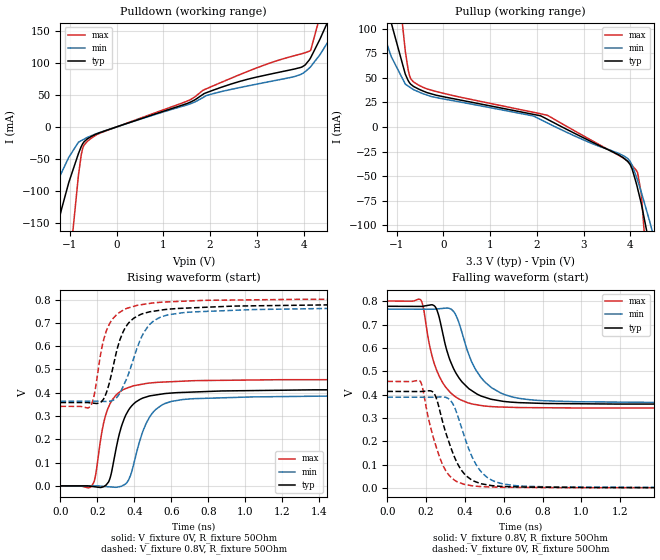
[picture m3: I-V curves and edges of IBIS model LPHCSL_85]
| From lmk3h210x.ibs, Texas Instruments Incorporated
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[Model]   LPHCSL_85
Model_type   Output
Polarity   Non-Inverting
Vmeas = 0.375
Vref = 0
Cref = 2pF
Rref = 100000
|   typ   min   max
C_comp   2.5pF   2pF   3pF
[Voltage Range]   3.3   3.135   3.465
[Temperature Range]   45   125   -40
[Pullup Reference]   3.3   3.135   3.465
[Pulldown Reference]   -0   -0   -0
[Power Clamp Reference]   3.3   3.135   3.465
[GND Clamp Reference]   0   0   0
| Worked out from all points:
|   slope of the pulldown table from 0 to 0.495 V, typ, clamps not added: 40.7 ohm
|   slope of the pullup table from 0 to 0.495 V, typ, clamps not added: 107 ohm
|   falling waveform, V_fixture 0.8V, R_fixture 50Ohm: 20-80 % time 123ps typ, 139ps min, 102ps max; typ from 0.779 V to 0.358 V
|   rising waveform, V_fixture 0V, R_fixture 50Ohm: 20-80 % time 90.9ps typ, 105ps min, 78.8ps max; typ from 0 V to 0.414 V
|   rising waveform, V_fixture 0.8V, R_fixture 50Ohm: 20-80 % time 99.8ps typ, 126ps min, 83.7ps max; typ from 0.358 V to 0.779 V
|   falling waveform, V_fixture 0V, R_fixture 50Ohm: 20-80 % time 106ps typ, 113ps min, 93.7ps max; typ from 0.414 V to 0 V
[Pulldown]
|   Voltage   I(typ)   I(min)   I(max)
-3.3V     -900mA     -529.4mA   -2.692A
-1.944V   -397.8mA   -215.8mA   -1.204A
-1.251V   -154.5mA   -84.31mA   -452.1mA
-1.023V   -86.95mA   -47.54mA   -227.5mA
-726mV    -26.52mA   -20.29mA   -33.92mA
-438.9mV  -11.27mA   -10.73mA   -12.68mA
3.977V    93.87mA    83.19mA    114.5mA
4.155V    108.2mA    94.14mA    119.8mA
4.353V    137mA      112.7mA    173mA
4.6V      177.5mA    141.8mA    276.7mA
4.927V    242.4mA    186.9mA    427.5mA
6.6V      632.4mA    489.5mA    1.311A
[Pullup]
|   Voltage   I(typ)   I(min)   I(max)
-3.3V     605.2mA    434.6mA    1.355A
-1.617V   212.4mA    144.7mA    463.6mA
-1.112V   105.1mA    71.14mA    210.1mA
-815.1mV  53.58mA    43.48mA    76.96mA
-726mV    44.97mA    40.66mA    52.4mA
-627mV    40.85mA    37.62mA    45.33mA
2.224V    7.749mA    4.058mA    11.86mA
3.937V    -34.84mA   -31.89mA   -34.65mA
4.155V    -62.59mA   -54.39mA   -46.61mA
4.372V    -111.3mA   -89.19mA   -155mA
4.491V    -145.8mA   -109.7mA   -248.9mA
6.6V      -933.8mA   -596.3mA   -2.548A
[Ramp]
R_load = 50
|   typ   min   max
dV/dt_r   0.248241/9.07181e-11   0.233324/1.04843e-10   0.27405/7.87855e-11
dV/dt_f   0.252877/1.21232e-10   0.242002/1.38069e-10   0.276271/1.01591e-10
[Falling Waveform]
V_fixture = 0.8V
V_fixture_min = 0.8V
V_fixture_max = 0.8V
R_fixture = 50Ohm
C_fixture = 0F
|   Time   V(typ)   V(min)   V(max)
0s        779.3mV    767mV      801.9mV
173.6ps   778.7mV    766.7mV    804.9mV
250.7ps   771.7mV    767.4mV    512.1mV
329.3ps   534.8mV    766.9mV    405.7mV
385.6ps   453.9mV    663.2mV    375.1mV
436.4ps   416.5mV    537.1mV    360.2mV
493.8ps   391.2mV    462.4mV    352mV
659.2ps   366.7mV    387.3mV    345.2mV
978.6ps   361mV      369.6mV    342.9mV
5ns       357.8mV    363.7mV    341.5mV
[Rising Waveform]
V_fixture = 0V
V_fixture_min = 0V
V_fixture_max = 0V
R_fixture = 50Ohm
C_fixture = 0F
|   Time   V(typ)   V(min)   V(max)
0s        161.5uV    251.5uV    87.97uV
173.6ps   -2.622mV   115.8uV    5.086mV
246.1ps   2.961mV    -2.859mV   306.9mV
271ps     40.38mV    -4.434mV   356.5mV
299.8ps   155.2mV    -5.936mV   389.1mV
368.1ps   325mV      24.64mV    422.2mV
465.5ps   382.2mV    271.2mV    440mV
549.7ps   394.6mV    347.8mV    445.6mV
720.7ps   403.1mV    374.4mV    451.7mV
5ns       413.9mV    389.1mV    456.8mV
[Rising Waveform]
V_fixture = 0.8V
V_fixture_min = 0.8V
V_fixture_max = 0.8V
R_fixture = 50Ohm
C_fixture = 0F
|   Time   V(typ)   V(min)   V(max)
0s        357.8mV    363.7mV    341.5mV
161ps     356.6mV    364mV      341mV
184.3ps   354.7mV    364mV      396.9mV
232.7ps   372.1mV    362.8mV    624.3mV
296.5ps   553.1mV    373.4mV    728.8mV
368.6ps   699.3mV    481.9mV    764.5mV
436.4ps   736.9mV    635.7mV    777.8mV
493.8ps   748.8mV    701.5mV    784.8mV
1.044ns   773.1mV    757.1mV    798.9mV
5ns       779.2mV    766.9mV    801.9mV
[Falling Waveform]
|Gnd
V_fixture = 0V
V_fixture_min = 0V
V_fixture_max = 0V
R_fixture = 50Ohm
C_fixture = 0F
|   Time   V(typ)   V(min)   V(max)
0s        414mV      389.2mV    456.9mV
167.9ps   413.4mV    389mV      459.1mV
232.7ps   412.7mV    388.9mV    228.6mV
281.9ps   292.8mV    390.5mV    105.1mV
335.6ps   153.7mV    363.4mV    39.6mV
385.6ps   71.4mV     250.1mV    18.19mV
438.8ps   32.17mV    129.2mV    8.673mV
536.7ps   9.866mV    33.6mV     3.873mV
720.7ps   3.187mV    6.643mV    1.869mV
5ns       160.8uV    251.3uV    87.05uV
